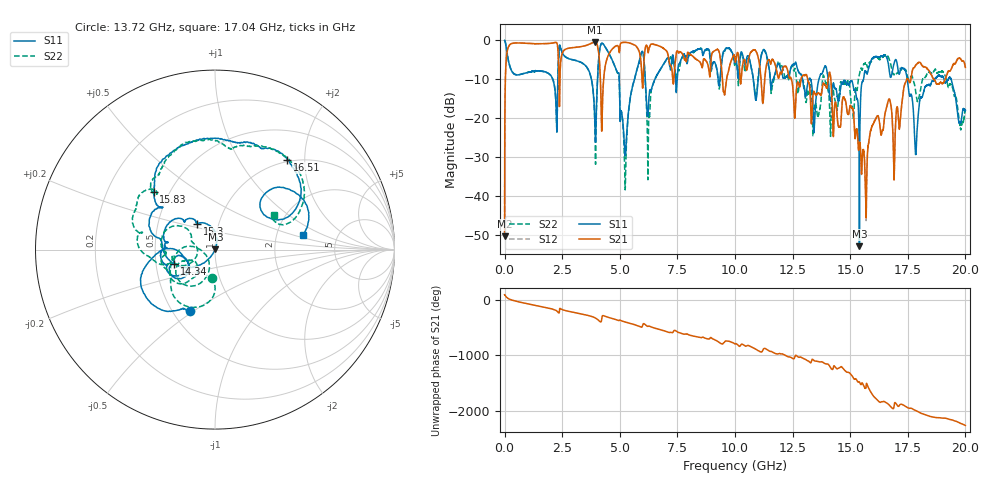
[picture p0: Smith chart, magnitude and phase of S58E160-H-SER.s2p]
!{S58E160}
!Johanson Technology Inc.
!www.johansontechnology.com
!Test Board Conditions:
!Substrate Type  RO4350B
!Substrate Thickness  60 mil
!Substrate Dk  3.66
!TL Type: GCPW
!TL Trace Width  115 mil
!TL Gap  52 mil
!Electrode orientation  Horizontal
!DUT TOPOLOGY	SERIES
!Mounting Pad LxW  55x428 mil
! Created Wed Apr 14 11:22:14 2021
# mhz S ma R 50
! 2 Port Network Data from SP1.SP block
! freq  magS11  angS11  magS21  angS21  magS12  angS12  magS22  angS22
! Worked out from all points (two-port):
!   20001 points, 300 kHz to 20 GHz, reference 50 ohm
!   highest |S21| = -0.41 dB at 3.916 GHz (marker M1); lowest = -50.4 dB at 300 kHz (marker M2)
!   |S21| within 3 dB of the highest: 95.29 MHz to 2.323 GHz (2.228 GHz wide, 184 % of centre); 2.493 GHz to 4.09 GHz (1.596 GHz wide, 48.5 % of centre)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
!   lowest |S11| = -52.9 dB at 15.4 GHz (marker M3), VSWR 1.00, Z = 50.2 + j0.0722 ohm
!   |S11| at or under -10 dB: 4.978 GHz to 5.637 GHz (659.2 MHz wide, 12.4 % of centre); 14.05 GHz to 15.58 GHz (1.53 GHz wide, 10.3 % of centre); 17.48 GHz to 18.66 GHz (1.181 GHz wide, 6.54 % of centre)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
!   |S22| runs from -38.4 to 0.0 dB; largest |S21 - S12| = 0.0094
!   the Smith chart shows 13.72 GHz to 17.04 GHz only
!   S11 on the Smith chart (normalised r, x): 13.72 GHz: 0.61, -0.48; 14.34 GHz: 0.62, -0.10; 15.3 GHz: 0.79, +0.24; 15.83 GHz: 0.41, +0.34; 16.51 GHz: 0.97, +1.65; 17.04 GHz: 2.81, +0.62
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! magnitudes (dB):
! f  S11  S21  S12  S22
! 300 kHz  0.0  -50.4  -50.3  0.0
! 222.3 MHz  -6.6  -1.1  -1.1  -6.5
! 3.334 GHz  -5.7  -1.6  -1.6  -5.7
! 3.916 GHz  -20.6  -0.4  -0.4  -21.7
! 4.234 GHz  -0.7  -19.2  -19.2  -0.7
! 5.229 GHz  -29.5  -0.5  -0.5  -37.6
! 5.91 GHz  -3.8  -5.1  -5.1  -3.7
! 6.23 GHz  -19.0  -3.1  -3.1  -29.8
! 6.667 GHz  -8.3  -1.3  -1.3  -8.3
! 10 GHz  -5.5  -5.1  -5.1  -6.1
! 13.33 GHz  -11.6  -20.0  -19.9  -15.1
! 13.72 GHz  -8.6  -14.0  -14.1  -16.1
! 14.34 GHz  -12.4  -16.1  -16.0  -15.4
! 15.3 GHz  -15.1  -22.9  -23.0  -12.8
! 15.4 GHz  -52.9  -26.5  -26.7  -8.8
! 15.83 GHz  -6.6  -25.2  -25.4  -5.7
! 16.51 GHz  -3.9  -19.0  -18.9  -3.8
! 16.67 GHz  -6.5  -15.2  -15.2  -4.4
! 17.04 GHz  -6.1  -17.1  -17.0  -8.4
! 17.85 GHz  -29.3  -6.3  -6.3  -13.4
! 18.79 GHz  -9.1  -11.2  -11.2  -8.4
! 20 GHz  -18.0  -6.9  -6.9  -17.6
